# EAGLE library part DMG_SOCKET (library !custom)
DMG Socket 32 Pin Cartridge Socket used in DMG-01
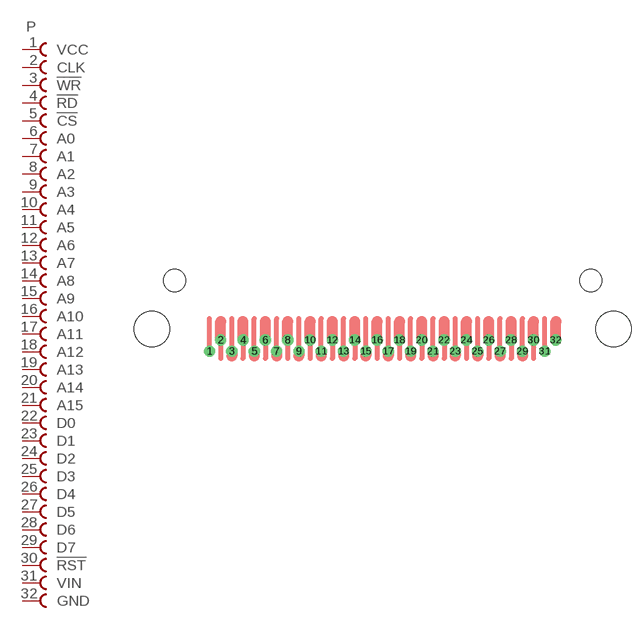
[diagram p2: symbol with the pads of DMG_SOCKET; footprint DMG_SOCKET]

Designator prefix P

## DMG_SOCKET  [DMG_SOCKET]
1  VCC  pas
2  CLK  pas
3  !WR  pas
4  !RD  pas
5  !CS  pas
6  A0  pas
7  A1  pas
8  A2  pas
9  A3  pas
10  A4  pas
11  A5  pas
12  A6  pas
13  A7  pas
14  A8  pas
15  A9  pas
16  A10  pas
17  A11  pas
18  A12  pas
19  A13  pas
20  A14  pas
21  A15  pas
22  D0  pas
23  D1  pas
24  D2  pas
25  D3  pas
26  D4  pas
27  D5  pas
28  D6  pas
29  D7  pas
30  !RST  pas
31  VIN  pas
32  GND  pas

## Footprint DMG_SOCKET (pad centres in mm)
drill 1 pad 1.5: 1 -23.25,-9.5; 2 -21.75,-8; 3 -20.25,-9.5; 4 -18.75,-8; 5 -17.25,-9.5; 6 -15.75,-8; 7 -14.25,-9.5; 8 -12.75,-8; 9 -11.25,-9.5; 10 -9.75,-8; 11 -8.25,-9.5; 12 -6.75,-8; 13 -5.25,-9.5; 14 -3.75,-8; 15 -2.25,-9.5; 16 -0.75,-8; 17 0.75,-9.5; 18 2.25,-8; 19 3.75,-9.5; 20 5.25,-8; 21 6.75,-9.5; 22 8.25,-8; 23 9.75,-9.5; 24 11.25,-8; 25 12.75,-9.5; 26 14.25,-8; 27 15.75,-9.5; 28 17.25,-8; 29 18.75,-9.5; 30 20.25,-8; 31 21.75,-9.5; 32 23.25,-8
hole 3 at -27.925,0
hole 3 at 27.925,0
hole 4.75 at -31,-6.5
hole 4.75 at 31,-6.5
